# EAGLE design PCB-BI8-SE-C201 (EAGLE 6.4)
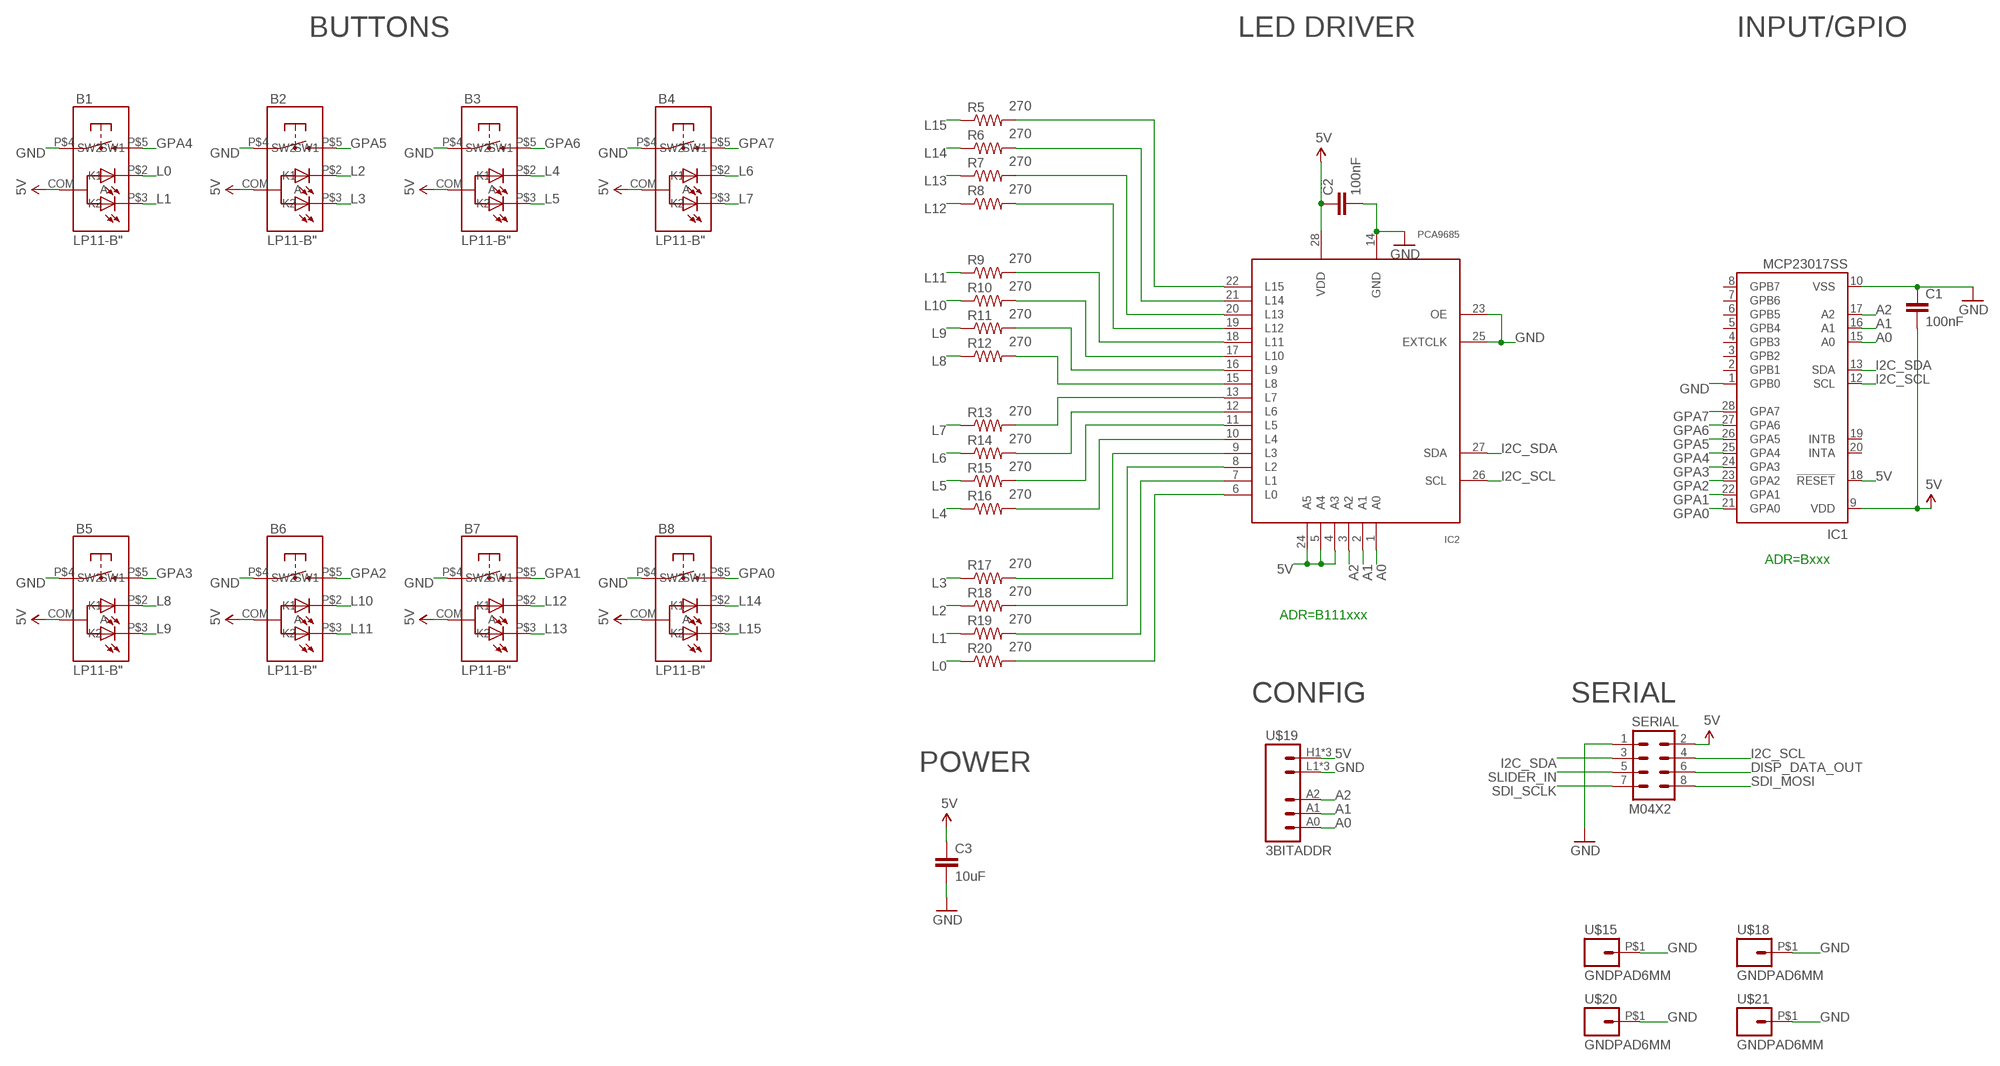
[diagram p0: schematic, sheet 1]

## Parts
B1  LP11-B"  [LP11]
B2  LP11-B"  [LP11]
B3  LP11-B"  [LP11]
B4  LP11-B"  [LP11]
B5  LP11-B"  [LP11]
B6  LP11-B"  [LP11]
B7  LP11-B"  [LP11]
B8  LP11-B"  [LP11]
C1  100nF  CAP0603-CAP  [0603-CAP]
C2  100nF  CAP0603-CAP  [0603-CAP]
C3  10uF  CAP0805  [0805]
IC1  MCP23017SS  [SSOP28]
IC2  PCA9685  [TSSOP28]
R5  270  RESISTOR0603-RES  [0603-RES]
R6  270  RESISTOR0603-RES  [0603-RES]
R7  270  RESISTOR0603-RES  [0603-RES]
R8  270  RESISTOR0603-RES  [0603-RES]
R9  270  RESISTOR0603-RES  [0603-RES]
R10  270  RESISTOR0603-RES  [0603-RES]
R11  270  RESISTOR0603-RES  [0603-RES]
R12  270  RESISTOR0603-RES  [0603-RES]
R13  270  RESISTOR0603-RES  [0603-RES]
R14  270  RESISTOR0603-RES  [0603-RES]
R15  270  RESISTOR0603-RES  [0603-RES]
R16  270  RESISTOR0603-RES  [0603-RES]
R17  270  RESISTOR0603-RES  [0603-RES]
R18  270  RESISTOR0603-RES  [0603-RES]
R19  270  RESISTOR0603-RES  [0603-RES]
R20  270  RESISTOR0603-RES  [0603-RES]
SERIAL  M04X2  [2X4]
U$15  GNDPAD6MM  [3.2MMPAD6MM]
U$18  GNDPAD6MM  [3.2MMPAD6MM]
U$19  3BITADDR  [3BITADDR]
U$20  GNDPAD6MM  [3.2MMPAD6MM]
U$21  GNDPAD6MM  [3.2MMPAD6MM]

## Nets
5V [Power]: B1.COM(A) B2.COM(A) B3.COM(A) B4.COM(A) B5.COM(A) B6.COM(A) B7.COM(A) B8.COM(A) C1.2 C2.1 C3.1 IC1.9(VDD) IC1.18(!RESET) IC2.4(A3) IC2.5(A4) IC2.24(A5) IC2.28(VDD) SERIAL.2 U$19.H1(VCC) U$19.H2(VCC) U$19.H3(VCC)
A0: IC1.15(A0) IC2.1(A0) U$19.A0
A1: IC1.16(A1) IC2.2(A1) U$19.A1
A2: IC1.17(A2) IC2.3(A2) U$19.A2
DISP_DATA_OUT: SERIAL.6
GND [Power]: B1.P$4(SW1) B2.P$4(SW1) B3.P$4(SW1) B4.P$4(SW1) B5.P$4(SW1) B6.P$4(SW1) B7.P$4(SW1) B8.P$4(SW1) C1.1 C2.2 C3.2 IC1.1(GPB0) IC1.10(VSS) IC2.14(GND) IC2.23(OE) IC2.25(EXTCLK) SERIAL.1 U$15.P$1 U$18.P$1 U$19.L1(GND) U$19.L2(GND) U$19.L3(GND) U$20.P$1 U$21.P$1
GPA0: B8.P$5(SW2) IC1.21(GPA0)
GPA1: B7.P$5(SW2) IC1.22(GPA1)
GPA2: B6.P$5(SW2) IC1.23(GPA2)
GPA3: B5.P$5(SW2) IC1.24(GPA3)
GPA4: B1.P$5(SW2) IC1.25(GPA4)
GPA5: B2.P$5(SW2) IC1.26(GPA5)
GPA6: B3.P$5(SW2) IC1.27(GPA6)
GPA7: B4.P$5(SW2) IC1.28(GPA7)
I2C_SCL: IC1.12(SCL) IC2.26(SCL) SERIAL.4
I2C_SDA: IC1.13(SDA) IC2.27(SDA) SERIAL.3
L0: B1.P$2(K1) R20.1
L1: B1.P$3(K2) R19.1
L2: B2.P$2(K1) R18.1
L3: B2.P$3(K2) R17.1
L4: B3.P$2(K1) R16.1
L5: B3.P$3(K2) R15.1
L6: B4.P$2(K1) R14.1
L7: B4.P$3(K2) R13.1
L8: B5.P$2(K1) R12.1
L9: B5.P$3(K2) R11.1
L10: B6.P$2(K1) R10.1
L11: B6.P$3(K2) R9.1
L12: B7.P$2(K1) R8.1
L13: B7.P$3(K2) R7.1
L14: B8.P$2(K1) R6.1
L15: B8.P$3(K2) R5.1
N$4: IC2.13(L7) R13.2
N$5: IC2.12(L6) R14.2
N$7: IC2.11(L5) R15.2
N$9: IC2.10(L4) R16.2
N$10: IC2.9(L3) R17.2
N$11: IC2.8(L2) R18.2
N$12: IC2.7(L1) R19.2
N$19: IC2.6(L0) R20.2
N$20: IC2.15(L8) R12.2
N$21: IC2.16(L9) R11.2
N$22: IC2.17(L10) R10.2
N$23: IC2.18(L11) R9.2
N$24: IC2.19(L12) R8.2
N$25: IC2.20(L13) R7.2
N$26: IC2.21(L14) R6.2
N$27: IC2.22(L15) R5.2
SDI_MOSI: SERIAL.8
SDI_SCLK: SERIAL.7
SLIDER_IN: SERIAL.5
Unconnected: IC1.2(GPB1) IC1.3(GPB2) IC1.4(GPB3) IC1.5(GPB4) IC1.6(GPB5) IC1.7(GPB6) IC1.8(GPB7) IC1.19(INTB) IC1.20(INTA)

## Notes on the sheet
- BUTTONS | LED DRIVER | INPUT/GPIO
- ADR=Bxxx
- ADR=B111xxx
- CONFIG | SERIAL
- POWER

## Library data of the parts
B1-B8 = SKAARHOJ:LP11-B
C1-C3 = SparkFun:CAP: Capacitor
IC1 = microchip:MCP23017: http://ww1.microchip.com/downloads/en/DeviceDoc/21952a.pdf Source: http://ww1.microchip.com/downloads/en/DeviceDoc/21952a.pdf; MF: MICROCHIP; MPN: MCP23017-E/SS; OC_FARNELL: 1467674; OC_NEWARK: 31K2960
IC2 = wsmith:PCA9685
R5-R20 = SparkFun:RESISTOR: Resistor
SERIAL = SparkFun:M04X2
U$15 U$18 U$20 U$21 = SKAARHOJ:GNDPAD
U$19 = SKAARHOJ:3BITADDR

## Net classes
0 default: width 0.203 mm, drill 0.406 mm, clearance 0.203 mm
1 Power: width 0.406 mm, drill 0.61 mm, clearance 0.203 mm

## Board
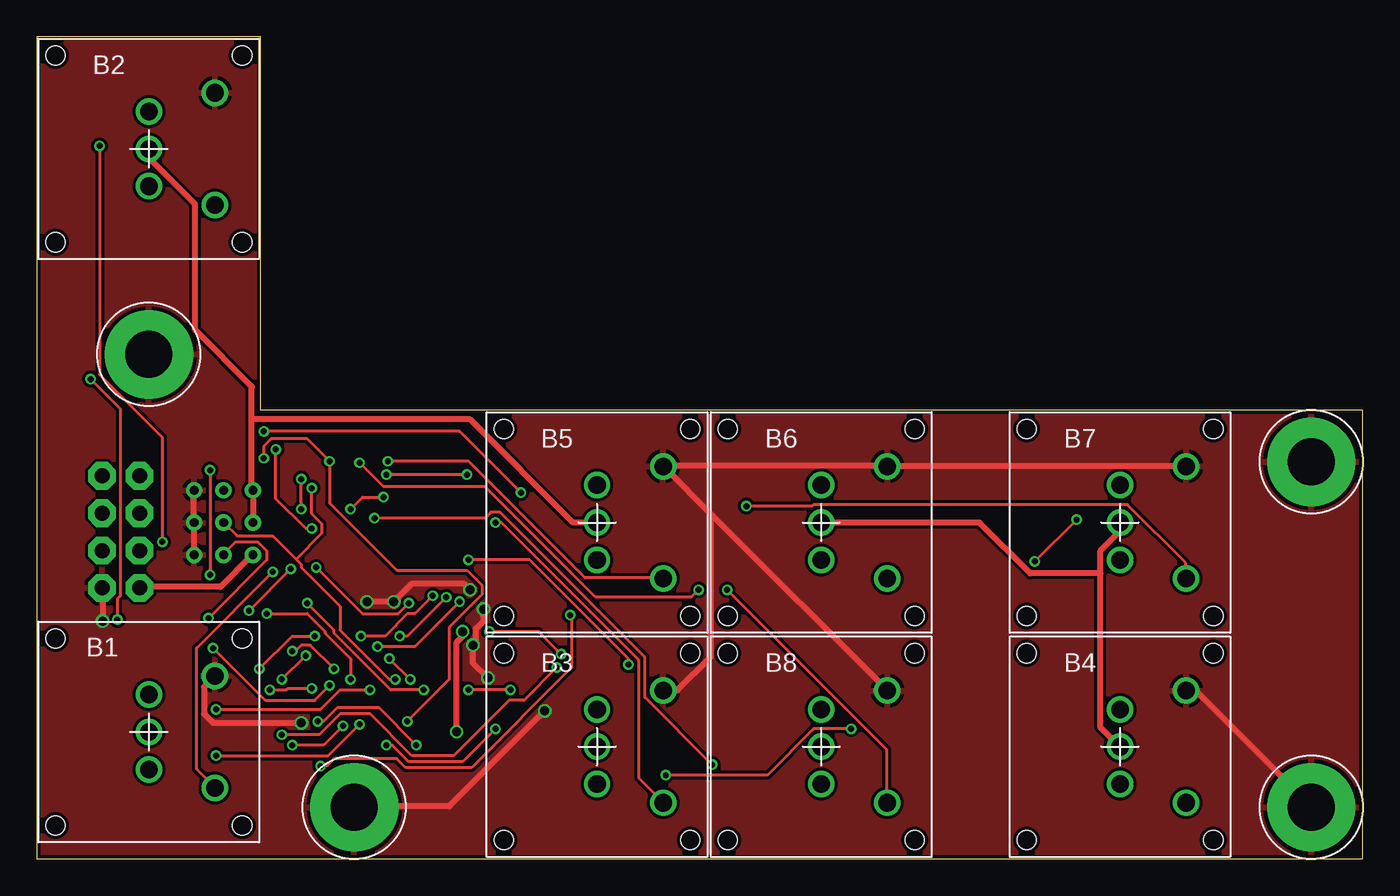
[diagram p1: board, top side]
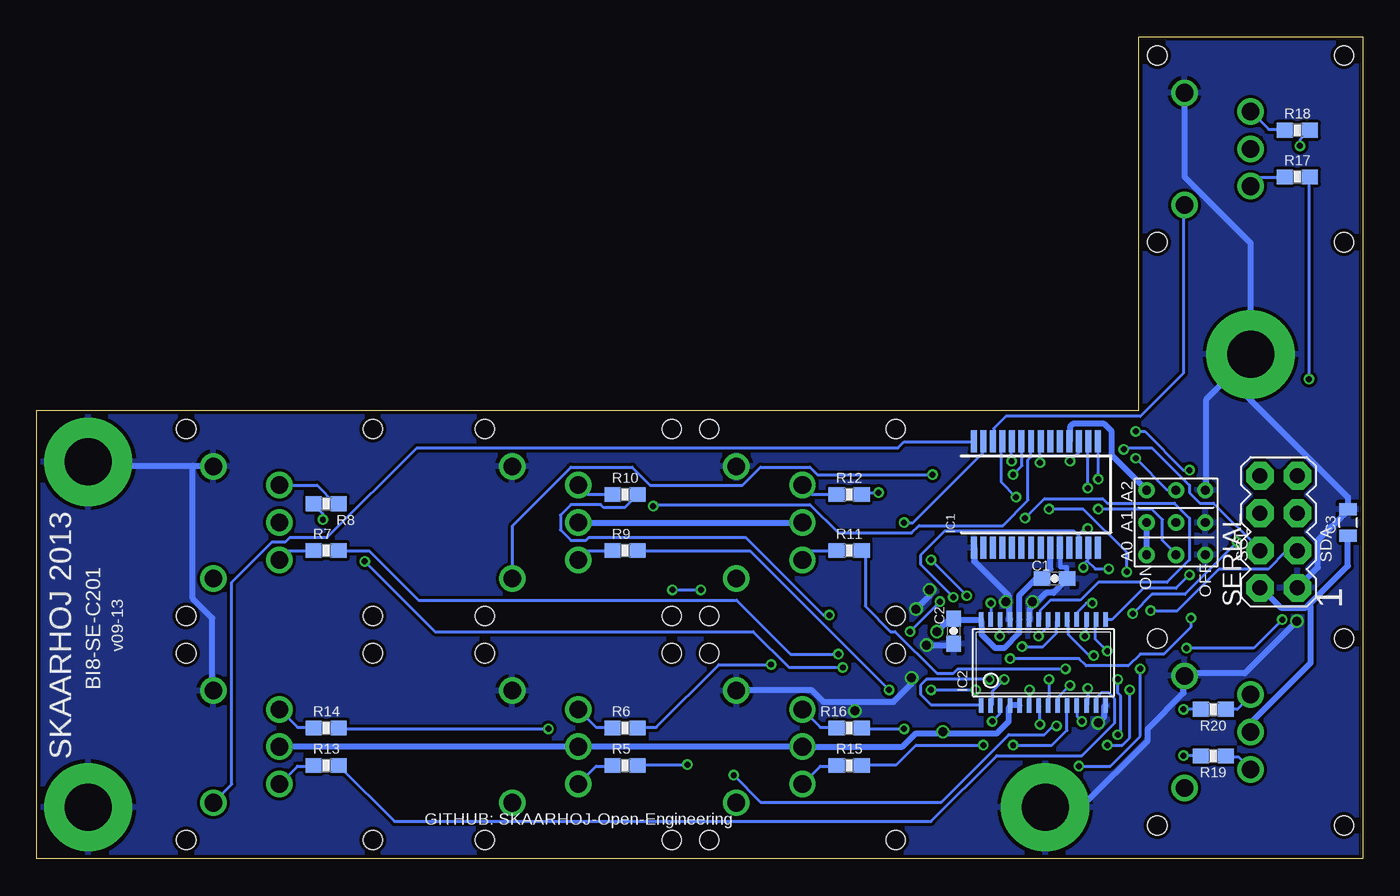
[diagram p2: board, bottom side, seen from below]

Size 90.17 x 55.88 mm. Coordinates in mm from the lower left corner, seen from the top.
Outline: 0,0 90.17,0 90.17,30.48 15.24,30.48 15.24,55.88 0,55.88 0,0
Copper layers (1*16): Top 0.035mm / dielectric 1.5mm / Bottom 0.035mm
Design rules "Fusion_eagle_rule_v1.1": minimum track width 6mil, minimum drill 12mil, track to track 6mil, track to pad 6mil, pad to pad 6mil, via to via 6mil, smd to smd 0mil, copper to edge 10mil, drill to drill 10mil, minimum pad ring 10mil, minimum via ring 6mil, stop-mask expansion 2mil, vias tented up to drill 100mil, thermal gap 10mil

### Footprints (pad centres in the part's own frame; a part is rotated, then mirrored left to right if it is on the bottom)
LP11 = drill 1.2: COM 0,0; P$2 0,2.54; P$3 0,-2.54; P$4 4.5,3.81; P$5 4.5,-3.81 | hole 1.3: -6.35,6.35; 6.35,6.35; 6.35,-6.35; -6.35,-6.35
0603-CAP = smd 1.1 x 1: 1 -0.85,0; 2 0.85,0
0805 = smd 0.8 x 1.2: 1 -0.9,0; 2 0.9,0
SSOP28 = smd 0.4 x 1.5: 1 -4.225,-3.625; 2 -3.575,-3.625; 3 -2.925,-3.625; 4 -2.275,-3.625; 5 -1.625,-3.625; 6 -0.975,-3.625; 7 -0.325,-3.625; 8 0.325,-3.625; 9 0.975,-3.625; 10 1.625,-3.625; 11 2.275,-3.625; 12 2.925,-3.625; 13 3.575,-3.625; 14 4.225,-3.625; 15 4.225,3.625; 16 3.575,3.625; 17 2.925,3.625; 18 2.275,3.625; 19 1.625,3.625; 20 0.975,3.625; 21 0.325,3.625; 22 -0.325,3.625; 23 -0.975,3.625; 24 -1.625,3.625; 25 -2.275,3.625; 26 -2.925,3.625; 27 -3.575,3.625; 28 -4.225,3.625
TSSOP28 = smd 0.305 x 0.991: 1 -4.225,-2.918; 2 -3.575,-2.918; 3 -2.925,-2.918; 4 -2.275,-2.918; 5 -1.625,-2.918; 6 -0.975,-2.918; 7 -0.325,-2.918; 8 0.325,-2.918; 9 0.975,-2.918; 10 1.625,-2.918; 11 2.275,-2.918; 12 2.925,-2.918; 13 3.575,-2.918; 14 4.225,-2.918; 15 4.225,2.918; 16 3.575,2.918; 17 2.925,2.918; 18 2.275,2.918; 19 1.625,2.918; 20 0.975,2.918; 21 0.325,2.918; 22 -0.325,2.918; 23 -0.975,2.918; 24 -1.625,2.918; 25 -2.275,2.918; 26 -2.925,2.918; 27 -3.575,2.918; 28 -4.225,2.918
0603-RES = smd 1.1 x 1: 1 -0.85,0; 2 0.85,0
2X4 = drill 1.016 pad 1.88 octagon: 1 -3.81,-1.27; 2 -3.81,1.27; 3 -1.27,-1.27; 4 -1.27,1.27; 5 1.27,-1.27; 6 1.27,1.27; 7 3.81,-1.27; 8 3.81,1.27
3.2MMPAD6MM = drill 3.2 pad 6: P$1 0,0
3BITADDR = drill 0.6: A0 -2.2,0; A1 0,0; A2 2.2,0; H1 -2.2,2; H2 0,2; H3 2.2,2; L1 -2.2,-2; L2 0,-2; L3 2.2,-2

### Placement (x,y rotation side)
B1  7.62,8.62 0 top
B2  7.62,48.26 0 top
B3  38.1,7.62 0 top
B4  73.66,7.62 0 top
B5  38.1,22.86 0 top
B6  53.34,22.86 0 top
B7  73.66,22.86 0 top
B8  53.34,7.62 0 top
C1  20.95,19.05 180 bottom
C2  27.81,15.47 270 bottom
C3  0.99,22.86 90 bottom
IC1  22.23,24.77 0 bottom
IC2  21.72,13.34 0 bottom
R5  50.16,6.35 0 bottom
R6  50.16,8.89 0 bottom
R7  70.48,20.95 0 bottom
R8  70.48,24.13 180 bottom
R9  50.16,20.95 0 bottom
R10  50.16,24.77 0 bottom
R11  34.92,20.95 0 bottom
R12  34.92,24.77 0 bottom
R13  70.48,6.35 0 bottom
R14  70.48,8.89 0 bottom
R15  34.92,6.35 0 bottom
R16  34.92,8.89 0 bottom
R17  4.45,46.35 0 bottom
R18  4.45,49.53 0 bottom
R19  10.16,6.99 180 bottom
R20  10.16,10.16 180 bottom
SERIAL  5.71,22.23 90 bottom
U$15  7.62,34.29 0 top
U$18  21.59,3.5 0 top
U$19  12.7,22.86 90 bottom
U$20  86.67,3.5 0 top
U$21  86.67,26.98 0 top

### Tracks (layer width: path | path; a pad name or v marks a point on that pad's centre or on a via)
5V  (via drill 0.61)
  Top 0.406: U$19.H2 14.73,22.86 14.73,24.99 U$19.H3 14.63,25.2 14.63,29.87 | B2.COM 7.62,47.65 10.77,44.5 10.77,35.97 14.63,32.11 14.63,29.87 | SERIAL.2 7.01,18.49 12.5,18.49 14.63,20.62 U$19.H1 | B7.COM 73.66,22.25 72.34,20.93 72.34,19.41 | 72.34,19.41 72.34,8.94 B4.COM | v28.96,15.44 28.96,15.14 28.55,14.73 v28.55,8.64 | B6.COM 64.11,22.86 67.56,19.41 72.34,19.41 | 14.63,29.87 29.46,29.87 36.47,22.86 B5.COM
  Bottom 0.406: 3.66,17.27 3.86,17.07 5.59,17.07 6.91,18.39 SERIAL.2 | 3.66,17.27 1.02,19.91 1.02,21.95 C3.1 | B1.COM 7.62,9.25 3.56,13.31 3.56,17.17 3.66,17.27 | U$19.H1 14.73,20.73 14.73,22.86 U$19.H2 | IC1.18 19.91,28.45 19.91,29.36 19.71,29.57 17.58,29.57 17.07,29.06 17.07,27.43 14.73,25.09 U$19.H3 | B6.COM B5.COM | IC1.9 21.23,21.13 21.23,19.71 21.74,19.2 C1.2 21.84,19 22.25,19 23.37,17.88 23.37,16.26 IC2.24 23.37,16.05 23.37,15.34 24.38,14.33 24.99,14.33 25.91,15.24 25.91,16.05 IC2.28 26.01,16.26 27.74,16.26 C2.1 27.94,16.26 28.14,16.26 v28.96,15.44 | IC2.5 23.37,10.46 23.98,10.46 IC2.4 24.08,10.26 24.08,9.35 24.89,8.53 28.55,8.53 | 28.55,8.53 30.38,8.53 31.29,7.62 B3.COM B8.COM B4.COM | v28.55,8.64 28.55,8.53
A0  (via drill 0.41)
  Top 0.203: v23.98,13.61 v25.4,12.19 | v11.68,16.36 15.65,20.32 15.65,20.93 15.04,21.54 13.51,21.54 12.7,20.73 U$19.A0 | v17.98,23.77 v17.98,25.81
  Bottom 0.203: v25.4,12.19 29.67,12.19 30.07,11.79 30.07,11.18 29.36,10.46 26.01,10.46 IC2.1 | v23.98,13.61 19.3,13.61 18.8,13.11 15.95,13.11 15.14,13.92 13.51,13.92 11.68,15.75 v11.68,16.36 | v17.98,25.81 17.98,28.35 IC1.15 | v17.98,23.77 14.33,23.77 13.61,23.06 13.61,21.64 12.7,20.73 U$19.A0
A1  (via drill 0.41)
  Top 0.203: v24.38,12.19 23.98,12.19 20.62,15.54 20.62,17.17 17.98,19.81 17.98,20.02 17.63,20.37 | 17.63,20.37 16.05,21.95 13.61,21.95 U$19.A1 | v18.69,25.2 18.69,23.47 19.41,22.76 19.41,22.15 17.63,20.37
  Bottom 0.203: v24.38,12.19 25.2,11.38 25.2,10.46 IC2.2 | v18.69,25.2 18.69,28.35 IC1.16
A2  (via drill 0.41)
  Top 0.203: v25.2,9.35 28.04,12.19 28.04,15.75 30.28,17.98 30.28,18.59 29.26,19.61 24.49,19.61 19.91,24.18 v19.91,27.03 18.39,28.55 15.95,28.55 15.44,28.04 v15.44,27.23
  Bottom 0.203: v25.2,9.35 24.69,9.86 24.69,10.36 IC2.3 | v19.91,27.03 19.3,27.64 19.3,28.35 IC1.17 | v15.44,27.23 13.31,25.09 12.7,25.09 U$19.A2
GND  (via drill 0.61)
  Top 0.406: v17.98,9.25 11.99,9.25 11.38,9.86 11.38,11.68 12.09,12.39 B1.P$4 | U$19.L1 10.67,20.73 10.67,22.86 U$19.L2 10.67,22.96 10.67,24.99 U$19.L3 | v4.47,16.15 4.47,18.39 SERIAL.1 | B4.P$4 78.23,11.38 78.84,11.38 86.67,3.56 U$20.P$1 | v22.45,17.48 v24.28,17.48 25.5,18.69 29.06,18.69 v29.46,18.29 | v30.68,12.29 29.67,13.31 v29.67,14.53 29.87,14.73 29.87,15.65 30.38,16.15 v30.38,16.97 | 45.92,23.37 42.67,26.62 B5.P$4 42.67,26.72 57.81,26.72 B6.P$4 58.01,26.72 78.13,26.72 B7.P$4 | 45.92,23.37 57.81,11.48 B8.P$4 | B3.P$4 42.67,11.48 43.59,11.48 45.82,13.72 45.82,23.27 45.92,23.37 | v34.54,10.06 28.04,3.56 21.64,3.56 U$18.P$1
  Bottom 0.305: IC1.10 20.57,21.14 20.57,19.81 20.11,19.81 C1.1
  Bottom 0.406: v17.98,9.25 17.58,9.65 17.58,10.36 IC2.14 | U$18.P$1 21.54,3.56 19.1,3.56 14.63,8.03 14.63,8.84 12.19,11.28 12.19,12.39 B1.P$4 11.99,12.6 8.03,12.6 v4.47,16.15 | SERIAL.1 3.05,19.81 3.05,21.64 1.02,23.67 C3.2 1.02,23.98 1.02,24.59 9.04,32.61 U$15.P$1 | U$15.P$1 7.62,41.86 12.09,46.33 12.09,52.02 B2.P$4 | U$19.L3 10.67,25.09 10.67,31.19 7.72,34.14 U$15.P$1 | 79.55,26.72 86.46,26.72 86.67,26.92 U$21.P$1 | 79.55,26.72 78.23,26.72 B7.P$4 | 79.55,26.72 79.55,17.68 78.23,16.36 78.23,11.48 B4.P$4 | 22.25,17.37 21.54,18.09 21.03,18.09 20.12,19 C1.1 | 22.25,17.37 22.66,16.97 22.66,16.26 IC2.23 | 24.08,17.48 24.08,17.88 26.42,20.22 26.42,21.13 IC1.1 | 24.08,17.48 24.08,16.26 IC2.25 | v22.45,17.48 22.35,17.48 22.25,17.37 | v24.28,17.48 24.08,17.48 | v29.67,14.53 27.84,14.53 C2.2 | v30.68,12.29 30.68,11.89 31.9,10.67 34.54,10.67 | 34.54,10.67 36.68,10.67 37.49,11.48 42.57,11.48 B3.P$4 | v29.46,18.29 29.46,17.88 v30.38,16.97 | 34.54,10.67 v34.54,10.06
  pour Top: 0,0 90.17,0 90.17,55.88 0,55.88
  pour Bottom: 0,0 90.17,0 90.17,55.88 0,55.88
GPA0  (via drill 0.41)
  Top 0.203: v21.95,26.92 23.57,25.3 30.48,25.3 38,17.78 44.5,17.78 v45.01,18.29 | v46.94,18.29 57.81,7.42 57.81,3.86 B8.P$5
  Bottom 0.203: v21.95,26.92 21.95,28.35 IC1.21 | v46.94,18.29 v45.01,18.29
GPA1  (via drill 0.41)
  Top 0.203: v48.26,23.98 52.73,23.98 52.83,24.08 74.17,24.08 78.13,20.12 78.13,19.1 B7.P$5
  Bottom 0.203: v48.26,23.98 48.16,24.08 37.59,24.08 35.66,22.15 30.68,22.15 30.18,22.66 24.49,22.66 22.76,24.38 22.76,27.13 22.55,27.33 22.55,28.35 IC1.22
GPA2  (via drill 0.41)
  Top 0.203: v29.26,26.11 v23.77,26.11
  Bottom 0.203: v23.77,26.11 23.16,26.72 23.16,28.35 IC1.23 | v29.26,26.11 37.08,26.11 37.59,26.62 40.95,26.62 42.16,25.4 48.46,25.4 49.68,26.62 53.85,26.62 57.81,22.66 57.81,19.1 B6.P$5
GPA3  (via drill 0.41)
  Top 0.203: v23.88,27.03 29.36,27.03 37.29,19.1 42.57,19.1 B5.P$5
  Bottom 0.203: v23.88,27.03 23.88,28.35 IC1.24
GPA4  (via drill 0.41)
  Top 0.203: v23.57,24.59 22.15,24.59 v21.34,23.77 | v16.05,19.51 10.87,14.33 10.87,6.1 12.09,4.88 B1.P$5
  Bottom 0.203: v23.57,24.59 24.59,25.6 24.59,28.35 IC1.25 | v21.34,23.77 19,23.77 16.05,20.83 v16.05,19.51
GPA5
  Bottom 0.203: IC1.26 25.09,28.45 25.09,29.26 24.28,30.07 15.14,30.07 12.19,33.02 12.19,44.4 B2.P$5
GPA6  (via drill 0.41)
  Top 0.203: v31.19,22.86 31.6,22.86 40.95,13.51 40.95,5.49 42.57,3.86 B3.P$5
  Bottom 0.203: v31.19,22.86 30.58,22.86 25.81,27.64 25.81,28.35 IC1.27
GPA7
  Bottom 0.203: IC1.28 26.52,28.35 31.19,28.35 31.6,27.94 64.31,27.94 70.41,21.84 72.95,21.84 73.25,21.54 74.17,21.54 76.91,18.8 76.91,5.08 78.13,3.86 B4.P$5
I2C_SCL  (via drill 0.41)
  Top 0.203: v24.69,15.14 25.2,15.14 v27.84,17.78 | v16.26,27.84 16.26,24.49 18.29,22.45 v18.69,22.45
  Bottom 0.203: v24.69,15.14 24.69,16.15 IC2.26 | v27.84,17.78 30.07,20.02 30.07,20.62 28.45,22.25 19.61,22.25 19.36,22 | 19.36,22 19.3,21.95 19.3,21.23 IC1.12 | v16.26,27.84 16.15,27.94 14.33,27.94 11.79,25.4 11.79,24.89 11.07,24.18 10.16,24.18 7.01,21.03 SERIAL.4 | v18.69,22.45 18.9,22.45 19.36,22
I2C_SDA  (via drill 0.41)
  Top 0.203: v25.3,17.37 24.59,16.66 22.15,16.66 v19,19.81 | v17.27,19.71 v14.43,16.87
  Bottom 0.203: v25.3,17.37 IC2.27 | v19,19.81 19,20.02 18.75,20.27 | 18.75,20.27 18.69,20.32 18.69,21.13 IC1.13 | v14.43,16.87 12.6,16.87 9.75,19.71 6.4,19.71 5.18,20.93 4.47,20.93 SERIAL.3 | v17.27,19.71 18.19,19.71 18.75,20.27
L0
  Bottom 0.203: R20.1 8.53,10.16 7.62,11.07 B1.P$2
L1
  Bottom 0.203: R19.1 9.25,6.91 8.43,6.91 7.62,6.1 B1.P$3
L2
  Bottom 0.203: B2.P$2 6.4,49.58 5.38,49.58 R18.1
L3
  Bottom 0.203: B2.P$3 7.01,46.33 5.38,46.33 R17.1
L4
  Bottom 0.203: B3.P$2 36.88,8.94 35.87,8.94 R16.1
L5
  Bottom 0.203: B3.P$3 36.88,6.3 35.87,6.3 R15.1
L6
  Bottom 0.203: B4.P$2 72.44,8.94 71.42,8.94 R14.1
L7
  Bottom 0.203: B4.P$3 72.44,6.3 71.42,6.3 R13.1
L8
  Bottom 0.203: B5.P$2 37.49,24.79 35.87,24.79 R12.1
L9
  Bottom 0.203: B5.P$3 37.49,20.93 35.87,20.93 R11.1
L10
  Bottom 0.203: B6.P$2 52.73,24.79 51.1,24.79 R10.1
L11
  Bottom 0.203: B6.P$3 52.73,20.93 51.1,20.93 R9.1
L12
  Bottom 0.203: B7.P$2 71.12,25.4 69.9,24.18 69.7,24.18 R8.1
L13
  Bottom 0.203: B7.P$3 73.05,20.93 71.42,20.93 R7.1
L14
  Bottom 0.203: B8.P$2 52.12,8.94 51.1,8.94 R6.1
L15
  Bottom 0.203: B8.P$3 52.12,6.3 51.1,6.3 R5.1
N$4
  Bottom 0.203: IC2.13 18.09,10.46 18.09,10.97 17.78,11.28 17.27,11.28 16.87,10.87 16.87,9.25 19.1,7.01 24.89,7.01 29.36,2.54 65.84,2.54 69.6,6.3 R13.2
N$5  (via drill 0.41)
  Top 0.203: v18.69,11.58 17.07,11.58 16.97,11.48 v15.85,11.48 | v17.37,7.72 19.51,7.72 v20.83,9.04 | v42.77,5.69 49.68,5.69 52.83,8.84 v55.37,8.84
  Bottom 0.203: v18.69,11.58 18.69,10.46 IC2.12 | v15.85,11.48 15.85,8.23 16.36,7.72 v17.37,7.72 | v20.83,9.04 21.03,9.04 21.64,8.43 24.08,8.43 28.65,3.86 40.95,3.86 v42.77,5.69 | v55.37,8.84 69.6,8.84 R14.2
N$7  (via drill 0.41)
  Top 0.203: v19.1,9.35 19.51,9.35 20.42,10.26 23.27,10.26 v25.81,7.72
  Bottom 0.203: v19.1,9.35 19.41,9.65 19.41,10.36 IC2.11 | v25.81,7.72 30.38,7.72 31.7,6.4 34.04,6.4 R15.2
N$9  (via drill 0.41)
  Top 0.203: v23.77,7.72 24.18,7.72 25.3,6.6 28.96,6.6 v31.19,8.84
  Bottom 0.203: v23.77,7.72 21.13,7.72 20.12,8.74 20.12,10.36 IC2.10 | v31.19,8.84 34.04,8.84 R16.2
N$10  (via drill 0.41)
  Top 0.203: v19.91,11.79 18.9,10.77 15.54,10.77 v11.99,14.33 | v5.49,16.26 5.49,17.68 5.69,17.88 5.69,30.58 v3.66,32.61
  Bottom 0.203: v19.91,11.79 20.73,10.97 20.73,10.46 IC2.9 | v11.99,14.33 7.42,14.33 v5.49,16.26 | v3.66,32.61 3.66,46.33 R17.2
N$11  (via drill 0.41)
  Top 0.203: v21.34,12.19 21.34,13.61 19.61,15.34 19.61,15.44 18.39,16.66 v15.65,16.66 | v8.53,21.54 8.53,28.65 4.27,32.92 v4.27,48.46
  Bottom 0.203: v21.34,12.19 21.34,10.46 IC2.8 | v15.65,16.66 14.33,17.98 12.09,17.98 v8.53,21.54 | v4.27,48.46 4.27,48.87 3.66,49.48 R18.2
N$12  (via drill 0.41)
  Top 0.203: v21.95,9.14 19.81,7.01 v12.19,7.01
  Bottom 0.203: v21.95,9.14 21.95,10.36 IC2.7 | v12.19,7.01 11.07,7.01 R19.2
N$19  (via drill 0.41)
  Top 0.203: v22.66,11.48 20.62,11.48 19.3,10.16 v12.19,10.16
  Bottom 0.203: v22.66,11.48 22.66,10.46 IC2.6 | R20.2 v12.19,10.16
N$20  (via drill 0.41)
  Top 0.203: v11.79,26.42 v11.79,19.3 | v15.44,29.06 28.75,29.06 v32.92,24.89
  Bottom 0.203: v11.79,19.3 12.7,18.39 14.94,18.39 17.07,16.26 17.48,16.26 IC2.15 | v11.79,26.42 12.19,26.42 14.83,29.06 v15.44,29.06 | v32.92,24.89 33.93,24.89 34.04,24.79 R12.2
N$21  (via drill 0.41)
  Top 0.203: v17.37,14.12 17.58,14.12 17.98,14.53 18.59,14.53 v20.22,12.9
  Bottom 0.203: v17.37,14.12 18.19,14.94 18.19,16.15 IC2.16 | v20.22,12.9 27.53,12.9 27.84,12.6 28.96,12.6 31.8,15.44 32.11,15.44 33.83,17.17 33.83,20.83 34.04,21.03 R11.2
N$22  (via drill 0.41)
  Top 0.203: v18.9,15.14 17.37,15.14 v15.14,12.9 | v19.3,6.3 19.71,6.3 20.22,6.81 24.49,6.81 25.09,6.2 29.57,6.2 36.37,13.01 36.37,16.46 v36.27,16.56
  Bottom 0.203: v18.9,15.14 18.8,15.24 18.8,16.15 IC2.17 | v15.14,12.9 15.14,8.33 17.17,6.3 v19.3,6.3 | v36.27,16.56 36.68,16.56 41.96,21.84 52.63,21.84 52.83,21.64 53.85,21.64 54.56,22.35 54.56,23.37 53.85,24.08 51.82,24.08 51.61,23.88 50.19,23.88 49.38,24.69 R10.2
N$23  (via drill 0.41)
  Top 0.203: v18.39,17.37 20.22,15.54 20.22,15.34 24.08,11.48 v26.31,11.48 | v32.21,11.48 v29.36,11.48
  Bottom 0.203: v18.39,17.37 18.8,17.37 19.41,16.76 19.41,16.26 IC2.18 | v29.36,11.48 v26.31,11.48 | v32.21,11.48 41.66,20.93 49.28,20.93 R9.2
N$24  (via drill 0.41)
  Top 0.203: v16.66,12.19 v18.29,13.82 | v16.66,8.43 19.2,8.43 20.62,9.86 22.66,9.86 25.5,7.01 28.35,7.01 32.11,10.77 33.12,10.77 v35.36,13.01 | v70.71,23.06 v67.87,20.22
  Bottom 0.203: v18.29,13.82 18.59,13.82 20.02,15.24 20.02,16.15 IC2.19 | v16.66,12.19 16.66,11.28 16.46,11.07 16.46,8.64 v16.66,8.43 | v35.36,13.01 39.01,13.01 41.45,15.44 63.09,15.44 v67.87,20.22 | v70.71,23.06 70.71,23.47 71.32,24.08 R8.2
N$25  (via drill 0.41)
  Top 0.203: v23.16,14.43 25.7,14.43 v28.75,17.48 | v30.79,15.44 34.14,15.44 v35.66,13.92
  Bottom 0.203: v23.16,14.43 21.74,14.43 20.83,15.34 20.83,16.15 IC2.20 | v30.79,15.44 v28.75,17.48 | v35.66,13.92 38.91,13.92 42.57,17.58 64.21,17.58 67.56,20.93 69.6,20.93 R7.2
N$26  (via drill 0.41)
  Top 0.203: v22.05,15.14 23.67,15.14 25.2,16.66 25.7,16.66 v26.92,17.88 | v29.36,20.32 33.53,20.32 40.23,13.61 v40.23,13.21
  Bottom 0.203: v22.05,15.14 21.44,15.75 21.44,16.15 IC2.21 | v29.36,20.32 v26.92,17.88 | v40.23,13.21 43.79,13.21 48.06,8.94 49.28,8.94 R6.2
N$27  (via drill 0.41)
  Top 0.203: v22.96,23.16 30.48,23.16 30.89,23.57 31.5,23.57 41.35,13.72 41.35,10.97 v45.92,6.4
  Bottom 0.203: v22.96,23.16 21.64,24.49 17.68,24.49 17.37,24.18 12.8,24.18 11.79,23.16 11.79,20.32 13.31,18.8 17.98,18.8 19.2,17.58 21.23,17.58 21.95,16.87 21.95,16.26 IC2.22 | v45.92,6.4 49.28,6.4 R5.2

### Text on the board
_bsilk: SKAARHOJ 2013 | SDA | SCL | BI8-SE-C201 | 1 | v09-13 | GITHUB: SKAARHOJ-Open-Engineering

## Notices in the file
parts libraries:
SparkFun: Licensing: CC v3.0 Share-Alike You are welcome to use this library for commercial purposes.
